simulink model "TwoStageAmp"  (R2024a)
settings: Solver=VariableStepAuto  StartTime=0.0  StopTime=1e-5  RelTol=1e-3  AbsTol=1e-3
libraries: fl_lib x10, nesl_utility x3, ee_lib x2

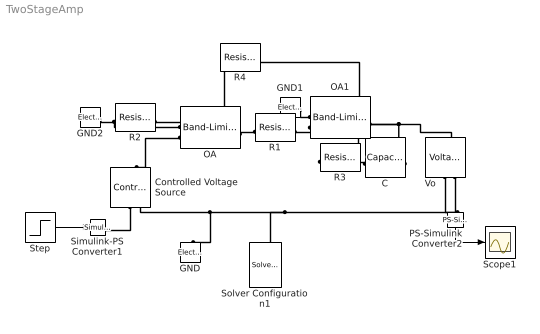
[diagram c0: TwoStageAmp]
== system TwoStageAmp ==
  C : fl_lib/Electrical/Electrical Elements/Capacitor  c=1 uF  r=1e-6 Ohm  g=0 1/Ohm  i_specify=off  i_priority=None  i=0 A  i_nominal_specify=off  i_nominal_value=1  i_nominal_unit=A  v_specify=off  v_priority=None  v=0 V  v_nominal_specify=off  v_nominal_value=1  v_nominal_unit=V  vc_specify=off  vc_priority=High  vc=0 V  vc_nominal_specify=off  vc_nominal_value=1  vc_nominal_unit=V
  Controlled Voltage Source : fl_lib/Electrical/Electrical Sources/Controlled Voltage Source
  GND : fl_lib/Electrical/Electrical Elements/Electrical Reference
  GND1 : fl_lib/Electrical/Electrical Elements/Electrical Reference
  GND2 : fl_lib/Electrical/Electrical Elements/Electrical Reference
  OA : ee_lib/Integrated Circuits/Band-Limited Op-Amp  A=5e5  Rin=1e6 Ohm  Rout=0 Ohm  Vmin=-15 V  Vmax=15 V  Vdotmax=1e7 V/s  f=20 Hz  V0=0 V
  OA1 : ee_lib/Integrated Circuits/Band-Limited Op-Amp  A=5e5  Rin=1e6 Ohm  Rout=0 Ohm  Vmin=-15 V  Vmax=15 V  Vdotmax=1e7 V/s  f=20 Hz  V0=0 V
  PS-Simulink Converter2 : nesl_utility/PS-Simulink Converter  PhysicalDomain=network_engine_domain  SubClassName=ps_output  LeftPortType=input  RightPortType=output  PseudoPeriodic=off  Frequencies=[]  VectorFormat=1-D array  Unit=inherit  AffineConversion=off
  R1 : fl_lib/Electrical/Electrical Elements/Resistor  R=1 kOhm  i_specify=off  i_priority=None  i=0 A  i_nominal_specify=off  i_nominal_value=1  i_nominal_unit=A  v_specify=off  v_priority=None  v=0 V  v_nominal_specify=off  v_nominal_value=1  v_nominal_unit=V
  R2 : fl_lib/Electrical/Electrical Elements/Resistor  R=1 kOhm  i_specify=off  i_priority=None  i=0 A  i_nominal_specify=off  i_nominal_value=1  i_nominal_unit=A  v_specify=off  v_priority=None  v=0 V  v_nominal_specify=off  v_nominal_value=1  v_nominal_unit=V
  R3 : fl_lib/Electrical/Electrical Elements/Resistor  R=1 kOhm  i_specify=off  i_priority=None  i=0 A  i_nominal_specify=off  i_nominal_value=1  i_nominal_unit=A  v_specify=off  v_priority=None  v=0 V  v_nominal_specify=off  v_nominal_value=1  v_nominal_unit=V
  R4 : fl_lib/Electrical/Electrical Elements/Resistor  R=499 kOhm  i_specify=off  i_priority=None  i=0 A  i_nominal_specify=off  i_nominal_value=1  i_nominal_unit=A  v_specify=off  v_priority=None  v=0 V  v_nominal_specify=off  v_nominal_value=1  v_nominal_unit=V
  Scope1 : Scope
  Simulink-PS Converter1 : nesl_utility/Simulink-PS Converter  PhysicalDomain=network_engine_domain  SubClassName=ps_input  LeftPortType=input  RightPortType=output  PseudoPeriodic=off  Frequencies=[]  NoiseDistribution=none  NoiseParameters=[]  Unit=1  AffineConversion=off  FilteringAndDerivatives=provide  SimscapeFilterOrder=1  InputFilterTimeConstant=0.001  UdotUserProvided=0
  Solver Configuration1 : nesl_utility/Solver Configuration  PhysicalDomain=network_engine_domain  SubClassName=solver  LeftPortType=input  RightPortType=generic  Tones=[]  Harmonics=[]  SimulateNoise=off  Profile=off  UseLocalSampling=off  EnableSwitchedLinearOptims=on  FrequencyDomain=off  UseCCode=off  RelTol=0.001  AbsTol=1e-06  MinStep=1e-09  ToWorkspace=off  RevertToSquareIcSolve=off  NumHomotopyIterations=100  PhasorMode=off  PhasorModeNumHarmonics=1  ConsistencySolver=NEWTON_FTOL  IndexReductionMethod=DerivativeReplacement  DoDC=on  ResidualTolerance=1e-09  ConsistencyTolSource=GLOBAL  ConsistencyAbsTol=0.001  ConsistencyRelTol=0.001  ConsistencyTolFactor=0.001  UseLocalSolver=off  LocalSolverChoice=NE_BACKWARD_EULER_ADVANCER  ResolveIndetEquations=on  FunctionEvalNumThread=1  LocalSolverSampleTime=0.001  DoFixedCost=off  MaxNonlinIter=3  MaxModeIter=2  ComputeImpulses=off  ImpulseIterations=2  LinearAlgebra=Sparse  LinearAlgebraNumThread=0  EquationFormulation=NE_TIME_EF  DelaysMemoryBudget=1024  AutomaticFiltering=on  FilteringTimeConstant=0.001  PartitionStorageMethod=AS_NEEDED  PartitionMemoryBudget=1024  PartitionMethod=FAST  MultibodyUseLocalSolver=off  MultibodyLocalSolverChoice=ODE1  MultibodyLocalSolverSampleTime=0.001
  Step : Step  SampleTime=0
  Vo : fl_lib/Electrical/Electrical Sensors/Voltage Sensor
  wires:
  Step/1 -> Simulink-PS Converter1/1
  PS-Simulink Converter2/1 -> Scope1/1
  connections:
  Vo/RConn2 -- GND/LConn1 -- Controlled Voltage Source/RConn2 -- Solver Configuration1/RConn1
  Vo/RConn1 -- PS-Simulink Converter2/LConn1
  Controlled Voltage Source/RConn1 -- Simulink-PS Converter1/RConn1
  OA/RConn1 -- R1/RConn1
  R2/LConn1 -- R4/RConn1 -- OA/LConn1
  OA/LConn2 -- Controlled Voltage Source/LConn1
  OA1/LConn2 -- R1/LConn1 -- R3/RConn1
  GND1/LConn1 -- OA1/LConn1
  C/RConn1 -- R3/LConn1
  OA1/RConn1 -- Vo/LConn1 -- R4/LConn1 -- C/LConn1
  GND2/LConn1 -- R2/RConn1
